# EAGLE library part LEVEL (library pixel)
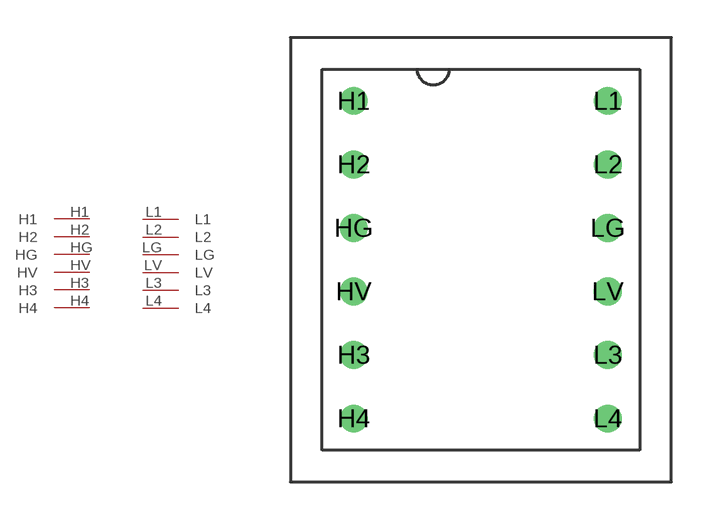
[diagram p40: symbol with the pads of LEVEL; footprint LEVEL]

Designator prefix -

## LEVEL  [LEVEL]
H1  H1
H2  H2
H3  H3
H4  H4
HG  HG
HV  HV
L1  L1
L2  L2
L3  L3
L4  L4
LG  LG
LV  LV

## Footprint LEVEL (pad centres in mm)
drill 0.6: H1 -5.08,6.35; H2 -5.08,3.81; H3 -5.08,-3.81; H4 -5.08,-6.35; HG -5.08,1.27; HV -5.08,-1.27; L1 5.08,6.35; L2 5.08,3.81; L3 5.08,-3.81; L4 5.08,-6.35; LG 5.08,1.27; LV 5.08,-1.27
